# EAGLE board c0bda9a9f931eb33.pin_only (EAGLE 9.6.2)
REV: B

Size 33.05 x 40.64 mm. Coordinates in mm from the lower left corner, seen from the top.
Outline: 2.56,0 arc-90 0.02,3.17 0.02,37.47 arc-90 2.56,40.64 30.5,40.64 arc-90 33.04,37.47 33.04,3.17 arc-90 30.5,0 2.56,0
Copper layers (1*16): Top 0.035mm / dielectric 1.5mm / Bottom 0.035mm
Design rules "adafruit 88": minimum track width 8mil, minimum drill 15.5mil, track to track 8mil, track to pad 8mil, pad to pad 8mil, via to via 8mil, smd to smd 8mil, copper to edge 10mil, drill to drill 8mil, minimum pad ring 10mil, minimum via ring 8mil, stop-mask expansion 2mil, vias tented up to drill 20mil, thermal gap 10mil
Holes 2 mm at 30.5,1.91 30.5,38.73 2.56,1.91 2.56,38.73

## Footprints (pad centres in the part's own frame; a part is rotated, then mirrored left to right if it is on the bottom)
SOLDERJUMPER_REFLOW_NOPASTE = smd 1.168 x 1.6: 1 -0.762,0; 2 0.762,0
0805-NO = smd 1.24 x 1.5: 1 -0.95,0; 2 0.95,0
0603-NO = smd 1.075 x 1: 1 -0.85,0; 2 0.85,0
1X04-CLEANBIG = drill 1.016 pad 1.778: 1 -3.81,0; 2 -1.27,0; 3 1.27,0; 4 3.81,0
JST_SH4 = smd 0.6 x 1.55: 1 -1.5,2.006; 2 -0.5,2.006; 3 0.5,2.006; 4 1.5,2.006 | smd 1.2 x 1.8: MT1 -2.8,-1.894; MT2 2.8,-1.894
SOD-323 = smd 1.35 x 0.8: A 1.27,0; C -1.27,0
SEGMENT_BICOL_BL-M12A883XX = drill 0.8 pad 1.676: 1 -13.97,-12; 2 -11.43,-12; 3 -8.89,-12; 4 -6.35,-12; 5 -3.81,-12; 6 -1.27,-12; 7 1.27,-12; 8 3.81,-12; 9 6.35,-12; 10 8.89,-12; 11 11.43,-12; 12 13.97,-12; 13 13.97,12; 14 11.43,12; 15 8.89,12; 16 6.35,12; 17 3.81,12; 18 1.27,12; 19 -1.27,12; 20 -3.81,12; 21 -6.35,12; 22 -8.89,12; 23 -11.43,12; 24 -13.97,12
SOP28_300MIL = smd 0.635 x 2.286: P$1 -8.255,-5.08; P$2 -6.985,-5.08; P$3 -5.715,-5.08; P$4 -4.445,-5.08; P$5 -3.175,-5.08; P$6 -1.905,-5.08; P$7 -0.635,-5.08; P$8 0.635,-5.08; P$9 1.905,-5.08; P$10 3.175,-5.08; P$11 4.445,-5.08; P$12 5.715,-5.08; P$13 6.985,-5.08; P$14 8.255,-5.08; P$15 8.255,5.08; P$16 6.985,5.08; P$17 5.715,5.08; P$18 4.445,5.08; P$19 3.175,5.08; P$20 1.905,5.08; P$21 0.635,5.08; P$22 -0.635,5.08; P$23 -1.905,5.08; P$24 -3.175,5.08; P$25 -4.445,5.08; P$26 -5.715,5.08; P$27 -6.985,5.08; P$28 -8.255,5.08
FIDUCIAL_1MM = smd 1 x 1: 1 0,0

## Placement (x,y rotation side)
A0  [SOLDERJUMPER_REFLOW_NOPASTE]  12.72,9.65 180 top
A1  [SOLDERJUMPER_REFLOW_NOPASTE]  12.72,7.49 180 top
A2  [SOLDERJUMPER_REFLOW_NOPASTE]  12.72,5.33 180 top
C1  10uF  [0805-NO]  19.07,33.02 180 top
C2  10uF  [0805-NO]  23.64,7.24 180 top
C3  1uF  [0603-NO]  8.15,6.99 180 top
CN1  1X4-CLEANBIG  [1X04-CLEANBIG]  16.53,38.73 0 top
CONN1  STEMMA_I2C_QT  [JST_SH4]  8.27,3.17 0 top
CONN2  STEMMA_I2C_QT  [JST_SH4]  24.78,3.17 0 top
D1  1N4148  [SOD-323]  18.56,6.99 270 top
E$2  [ADAFRUIT_3.5MM]  29.23,0.06 0 bottom
LED2  [SEGMENT_BICOL_BL-M12A883XX]  16.53,20.32 270 bottom
PLABEL0  [PLABEL0]  15.7,34.92 90 top
PLABEL1  [PLABEL1]  13.16,35.05 90 top
PLABEL2  [PLABEL2]  20.91,34.92 90 top
PLABEL3  [PLABEL3]  18.37,34.8 90 top
PLABEL4  [PLABEL4]  7.51,13.72 90 top
PLABEL5  [PLABEL5]  2.05,20.57 90 top
PLABEL6  [PLABEL6]  10.81,9.02 90 top
PLABEL7  [PLABEL7]  10.81,6.73 90 top
PLABEL8  [PLABEL8]  11.83,3.05 0 top
PLABEL9  [PLABEL9]  31.39,20.7 90 top
PLABEL10  [PLABEL10]  14.69,1.91 0 bottom
PLABEL11  [PLABEL11]  12.08,37.02 0 bottom
PLABEL12  [PLABEL12]  16.27,36.96 0 bottom
PLABEL13  [PLABEL13]  19.07,36.96 0 bottom
PLABEL14  [PLABEL14]  23.51,36.89 0 bottom
R1  10K  [0603-NO]  22.5,30.73 0 top
R2  10K  [0603-NO]  22.5,32.77 0 top
R3  47K  [0603-NO]  16.02,7.49 180 top
R4  47K  [0603-NO]  16.02,9.27 180 top
R5  47K  [0603-NO]  16.02,5.71 180 top
U2  28-SOIC  [SOP28_300MIL]  16.53,20.32 270 top
U$1  FIDUCIAL  [FIDUCIAL_1MM]  8.65,34.54 90 top
U$2  FIDUCIAL  [FIDUCIAL_1MM]  25.93,14.99 90 top
U$3  [ADAFRUIT_5MM]  13.99,0.13 0 top
U$4  [PCBFEAT-REV-040]  5.61,36.83 90 top

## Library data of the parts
A0 A1 A2 C1-C3 D1 E$2 R1-R5 U$3 U$4 = microbuilder
CN1 U$1 U$2 = adafruit
CONN1 CONN2 = adafruit_electromech; LCSC: C2845363
LED2 U2 = adafruit_display
PLABEL0 PLABEL1-PLABEL14 = pinguin

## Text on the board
bDocu: C | D | - | +
Pinguin_tBackup: SCL | SDA | GND | VCC | HT16K33 LED Backpack | 8x8 Bi-Color LED Matrix | from adafruit! | A0 | A1 | A2
Pinguin_bBackup: VCC | SCL | SDA | GND | 8x8 Bi-Color LED Matrix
